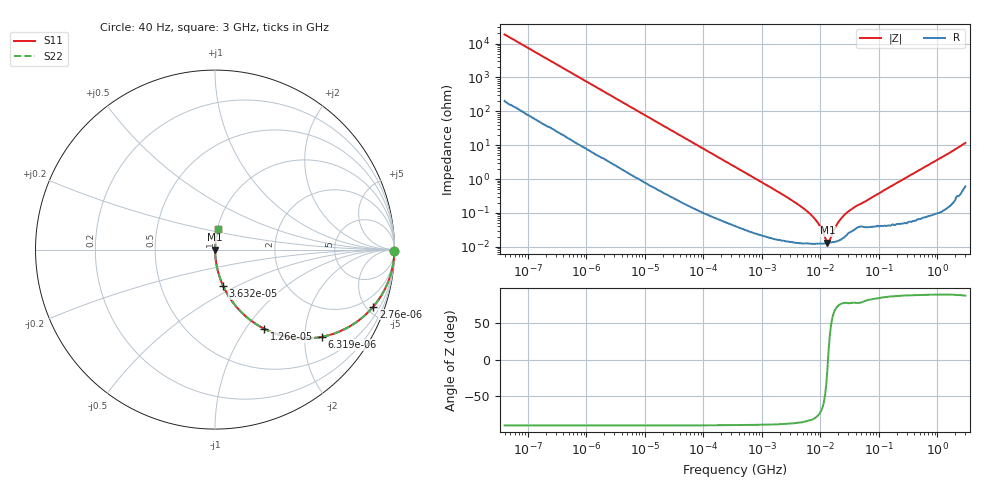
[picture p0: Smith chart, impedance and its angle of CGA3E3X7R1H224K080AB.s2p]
! S-parameter Generated by TDK Corporation
! Copyright(C) 2015 TDK Corporation.
! All Rights Reserved.
! TDK P/N: CGA3E3X7R1H224K080AB (Multilayer Ceramic Chip Capacitors)
! Property: C=220nF
! Size(LxWxT): 1.6x0.8x0.8mm, 0.063x0.031x0.031inches
! Model Type: s2p (Touchstone File Format Version 1.0)
! Frequency: DC=Yes Start=0.00004MHz Stop=3000MHz 396points Log-sweep
! Note: This model was converted from impedance.
! Model Generated on Jun. 23, 2015
! Hash(MD5):
! Port Assignments:
!  1 ---| |--- 2
! Applicable Conditions:
!  Temperature = 25 degC
!  DC Bias Voltage = 0 V
!  Small Signal Operation
! Terms and conditions regarding TDK Simulation Models
! (1)This simulation model is being provided solely for informational purposes. Please refer to the specifications of the products in terms of detailed characteristics of such products.
! (2)In no event shall TDK Corporation of any of its subsidiaries be liable for any loss or damage arising, directly or indirectly,
!  From any information contained in this simulation model, including, but not limited to loss or damages arising from any inaccuracies, omissions or errors in connection with such information.
! (3)Any and all copyrights on this simulation model are owned by TDK Corporation.
!  Duplication or redistribution of this simulation model without prior written permission from TDK Corporation is prohibited.
! (4)This simulation model is subject to any modification or change without any prior notice.
! (5)Neither TDK Corporation nor any of its subsidiaries shall make any warranty, express or implied,
!  Including but not limited to the correctness, implied warranties of merchantability and fitness for a particular purpose with respect to this simulation models.
! (6)The use of this simulation model shall be deemed to have consented to the terms and conditions hereof.
# MHz S MA R 50
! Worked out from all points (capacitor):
!   395 points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, 40 Hz to 3 GHz, reference 50 ohm
!   read as one part in series: C = 214 nF near 41.88 Hz
!   lowest |Z| = 13.1 mohm at 13.14 MHz (marker M1)
!   series resonance near 13.46 MHz, so ESL is about 650 pH
!   S11 on the Smith chart (normalised r, x): 40 Hz: open; 2.76 kHz: 1.06, -5.53; 6.319 kHz: 1.02, -2.43; 12.6 kHz: 1.01, -1.22; 36.32 kHz: 1.00, -0.43; 3 GHz: 1.01, +0.23
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4e-05  0.9999 -0.3  0.005383 89.1  0.005383 89.1  0.9999 -0.3
0.0002520917  0.9991 -1.9  0.03349 87.5  0.03349 87.5  0.9991 -1.9
0.000834128  0.9929 -6.3  0.1093 83.1  0.1093 83.1  0.9929 -6.3
0.002759985  0.9374 -19.8  0.3387 69.6  0.3387 69.6  0.9374 -19.8
0.006319477  0.7684 -39.2  0.6322 50.2  0.6322 50.2  0.7684 -39.2
0.01260356  0.5198 -58.1  0.849 31.3  0.849 31.3  0.5198 -58.1
0.01739424  0.4046 -65.5  0.9103 23.9  0.9103 23.9  0.4046 -65.5
0.03632493  0.209 -77.3  0.9756 12.1  0.9756 12.1  0.209 -77.3
0.09548642  0.08188 -84.6  0.9956 4.7  0.9956 4.7  0.08188 -84.6
0.3464102  0.02291 -87.7  0.9993 1.3  0.9993 1.3  0.02291 -87.7
2.748062  0.002832 -86.9  0.9999 0.2  0.9999 0.2  0.002832 -86.9
4.998775  0.001408 -84.8  0.9999 0.1  0.9999 0.1  0.001408 -84.8
7.22376  0.0008127 -81.3  0.9999 0.0  0.9999 0.0  0.0008127 -81.3
9.969551  0.0003898 -71.2  0.9999 0.0  0.9999 0.0  0.0003898 -71.2
13.14015  0.0001313 -13.1  0.9999 0.0  0.9999 0.0  0.0001313 -13.1
13.75903  0.0001342 11.8  0.9999 -0.0  0.9999 -0.0  0.0001342 11.8
18.98891  0.0004528 71.4  0.9999 -0.0  0.9999 -0.0  0.0004528 71.4
27.44099  0.0009755 77.3  0.9998 -0.1  0.9998 -0.1  0.0009755 77.3
39.65514  0.001543 77.3  0.9997 -0.1  0.9997 -0.1  0.001543 77.3
150.6385  0.005734 85.3  0.9995 -0.3  0.9995 -0.3  0.005734 85.3
994.0817  0.03676 86.4  0.9983 -2.1  0.9983 -2.1  0.03676 86.4
3000  0.1158 80.4  0.9873 -6.6  0.9873 -6.6  0.1158 80.4
